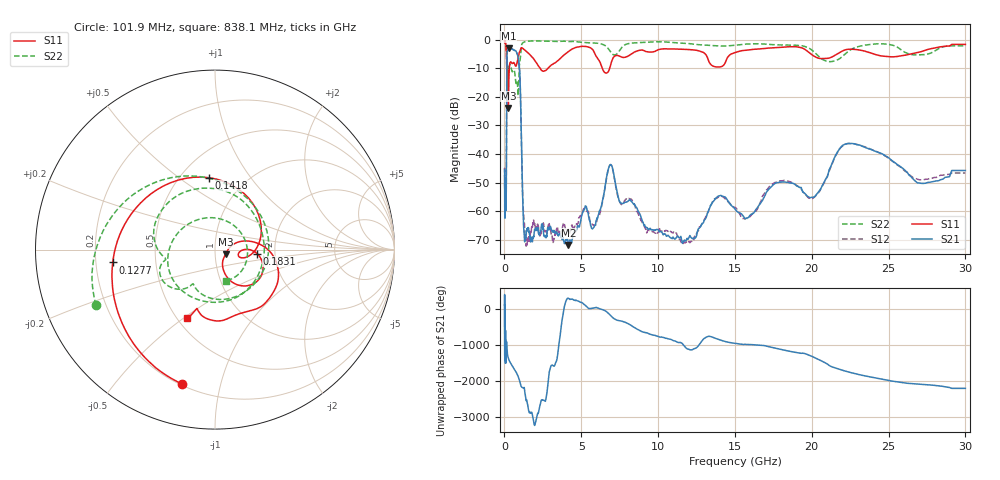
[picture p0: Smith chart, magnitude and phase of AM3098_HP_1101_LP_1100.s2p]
! Date/Time: Thu, Feb 28, 2019 8:45 AM
! Network Analyzer: Agilent Technologies E8364B Rev: A.07.50.67
! Sweep from 0.010 to 30.000 GHz, 1601 Points, Sweep Type: LOG
! Power Supply: 5.022 V, 0.002 A
# Hz S DB R 50
!freq MagS11 AngS11 MagS21 AngS21 MagS12 AngS12 MagS22 AngS22
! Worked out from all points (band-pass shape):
!   1601 points, 10 MHz to 30 GHz, reference 50 ohm
!   highest |S21| = -3.09 dB at 267.8 MHz (marker M1); lowest = -71.8 dB at 4.156 GHz (marker M2)
!   |S21| within 3 dB of the highest: 159.2 MHz to 887.4 MHz (728.1 MHz wide, 139 % of centre)
!   lowest |S11| = -23.9 dB at 253.4 MHz (marker M3), VSWR 1.14, Z = 56.1 - j2.83 ohm
!   |S11| at or under -10 dB: 148 MHz to 317.3 MHz (169.3 MHz wide, 72.8 % of centre); 2.322 GHz to 2.836 GHz (514.2 MHz wide, 19.9 % of centre); 6.363 GHz to 6.85 GHz (486.9 MHz wide, 7.37 % of centre)
!   |S22| runs from -19.5 to -0.5 dB; largest |S21 - S12| = 0.011
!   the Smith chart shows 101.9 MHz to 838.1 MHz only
!   S11 on the Smith chart (normalised r, x): 101.9 MHz: 0.21, -0.77; 127.7 MHz: 0.27, -0.06; 141.8 MHz: 0.68, +0.65; 183.1 MHz: 1.61, -0.08; 838.1 MHz: 0.56, -0.51
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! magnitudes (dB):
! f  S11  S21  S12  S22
! 10 MHz  -0.3  -45.4  -45.4  -0.6
! 38.04 MHz  -0.3  -60.8  -58.3  -0.8
! 101.9 MHz  -2.3  -59.4  -55.8  -2.7
! 127.7 MHz  -4.8  -40.8  -41.1  -6.2
! 141.8 MHz  -7.9  -17.7  -17.6  -10.5
! 144.7 MHz  -8.8  -14.3  -14.2  -10.7
! 183.1 MHz  -12.6  -4.1  -4.1  -10.6
! 253.4 MHz  -23.9  -3.1  -3.1  -11.1
! 267.8 MHz  -19.4  -3.1  -3.1  -10.9
! 550.5 MHz  -8.2  -3.5  -3.5  -10.8
! 838.1 MHz  -7.7  -5.1  -5.1  -14.7
! 1.009 GHz  -4.1  -13.0  -13.0  -7.6
! 1.295 GHz  -3.6  -69.4  -64.0  -0.8
! 2.084 GHz  -8.1  -66.3  -65.8  -0.5
! 4.156 GHz  -4.2  -71.8  -66.2  -0.6
! 5.959 GHz  -5.8  -63.4  -64.6  -1.2
! 6.855 GHz  -9.9  -43.9  -43.8  -3.9
! 7.926 GHz  -6.1  -56.8  -55.6  -1.6
! 11.83 GHz  -3.4  -70.1  -70.7  -1.4
! 20.1 GHz  -5.6  -55.1  -55.3  -4.1
! 22.56 GHz  -3.4  -36.3  -36.3  -3.5
! 30 GHz  -1.7  -45.7  -46.6  -2.2
